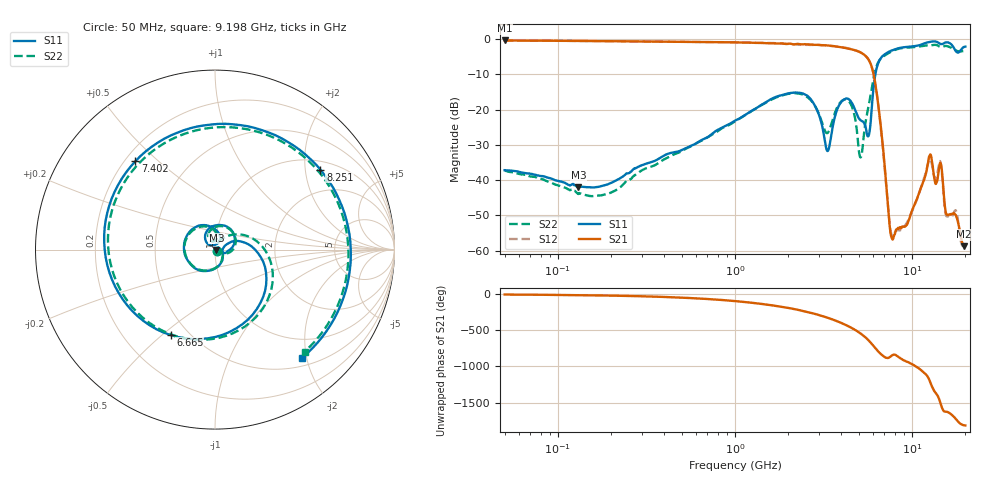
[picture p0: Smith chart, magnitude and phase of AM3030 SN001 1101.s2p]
# Hz S DB R 50
!freq MagS11 AngS11 MagS21 AngS21 MagS12 AngS12 MagS22 AngS22
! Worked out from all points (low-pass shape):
!   1601 points, 50 MHz to 20.05 GHz, reference 50 ohm
!   highest |S21| = -0.36 dB at 50 MHz (marker M1); lowest = -58.8 dB at 19.68 GHz (marker M2)
!   |S21| within 3 dB of the highest: start of sweep to 4.927 GHz
!   lowest |S11| = -42.1 dB at 130.5 MHz (marker M3), VSWR 1.02, Z = 50.7 - j0.276 ohm
!   |S11| at or under -10 dB: start of sweep to 6.213 GHz
!   |S22| runs from -44.6 to -1.6 dB; largest |S21 - S12| = 0.022
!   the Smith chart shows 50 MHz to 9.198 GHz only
!   S11 on the Smith chart (normalised r, x): 50 MHz: 1.03, -0.01; 6.665 GHz: 0.40, -0.53; 7.402 GHz: 0.24, +0.42; 8.251 GHz: 1.24, +2.42; 9.198 GHz: 0.63, -1.91
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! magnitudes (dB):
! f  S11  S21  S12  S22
! 50 MHz  -37.2  -0.4  -0.3  -37.3
! 130.5 MHz  -42.1  -0.5  -0.5  -43.9
! 135.9 MHz  -41.9  -0.5  -0.5  -43.9
! 369.6 MHz  -34.0  -0.7  -0.7  -35.1
! 1.005 GHz  -23.1  -0.9  -0.9  -23.3
! 2.722 GHz  -17.5  -1.5  -1.6  -17.7
! 3.333 GHz  -31.8  -1.8  -1.8  -26.6
! 4.316 GHz  -16.9  -2.6  -2.5  -17.3
! 5.127 GHz  -23.0  -3.7  -3.7  -33.5
! 5.694 GHz  -27.4  -5.8  -5.8  -18.9
! 6.207 GHz  -10.1  -12.6  -12.3  -8.9
! 6.665 GHz  -5.4  -24.5  -25.0  -5.5
! 7.402 GHz  -3.6  -50.6  -50.0  -3.9
! 8.251 GHz  -2.6  -53.9  -54.2  -2.8
! 9.198 GHz  -2.2  -53.1  -52.7  -2.4
! 12.69 GHz  -0.7  -32.7  -34.2  -1.7
! 13.63 GHz  -0.7  -41.1  -39.6  -1.6
! 14.47 GHz  -1.3  -35.0  -34.8  -2.2
! 15.66 GHz  -0.9  -49.7  -50.3  -1.9
! 17.72 GHz  -3.4  -50.0  -48.6  -3.2
! 19.68 GHz  -2.2  -58.8  -58.5  -3.3
! 20.05 GHz  -2.1  -58.4  -58.2  -3.3
